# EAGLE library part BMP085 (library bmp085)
BMP085 Digital pressure sensor
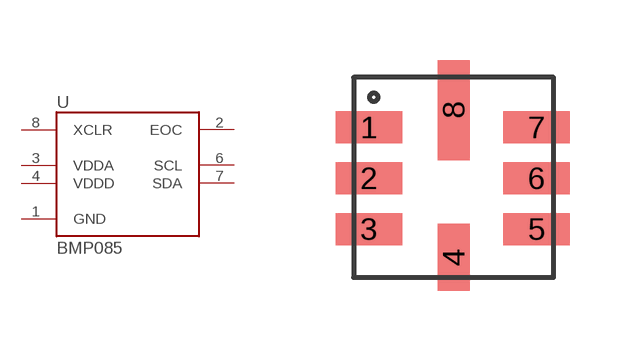
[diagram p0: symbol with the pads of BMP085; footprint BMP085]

Designator prefix -

## BMP085  [BMP085]
1  GND  pwr
2  EOC  out
3  VDDA  pwr
4  VDDD  pwr
5  NC  nc
6  SCL  in
7  SDA
8  XCLR  in

## Footprint BMP085 (pad centres in mm)
smd 1.67 x 0.8: 1 -2.159,1.206; 2 -2.159,-0.064; 3 -2.159,-1.333; 5 2.032,-1.333; 6 2.032,-0.064; 7 2.032,1.206
smd 0.8 x 1.67: 4 -0.04,-2.04
smd 0.8 x 2.5: 8 -0.04,1.643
